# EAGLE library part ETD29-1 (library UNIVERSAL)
Transformator ETD29
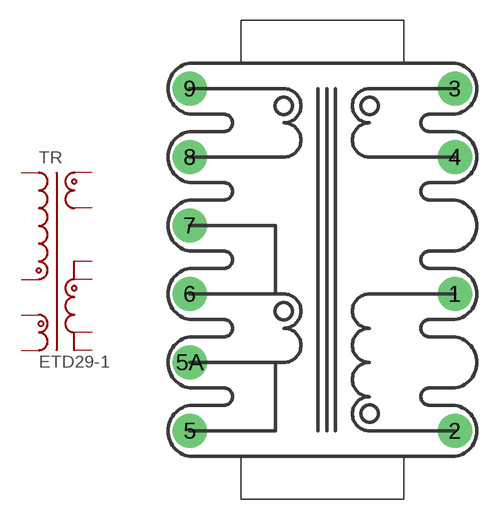
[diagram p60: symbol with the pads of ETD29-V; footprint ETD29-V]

Designator prefix TR

## ETD29-1 (TR: ETD29)  [ETD29-V]
1  1
2  2
3  3
4  4
5  5
5A  5A
6  6
7  7
8  8
9  9

## Footprint ETD29-V (pad centres in mm)
drill 0.8 pad 2.54: 1 19.685,10.16; 2 19.685,0; 3 19.685,25.4; 4 19.685,20.32; 5 0,0; 5A 0,5.08; 6 0,10.16; 7 0,15.24; 8 0,20.32; 9 0,25.4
